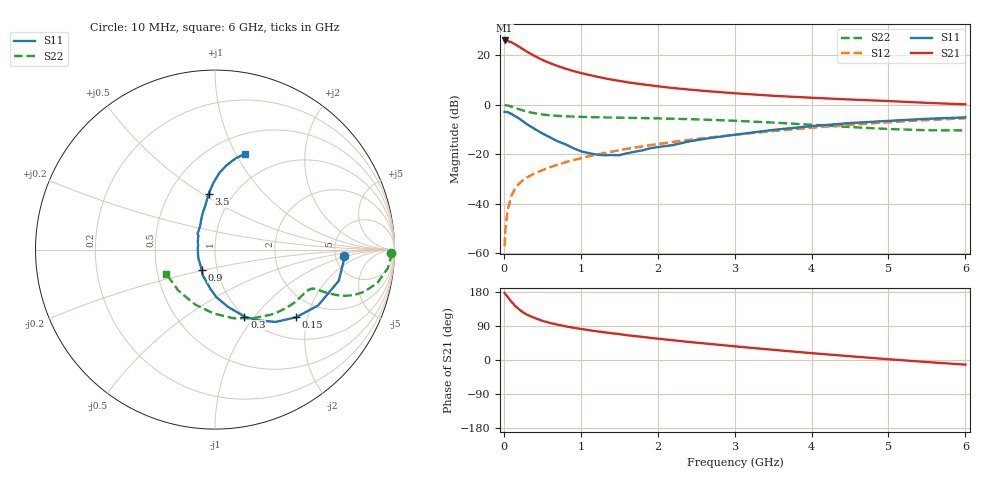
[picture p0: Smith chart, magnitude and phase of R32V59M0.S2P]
! SIEMENS Small Signal Semiconductors
! BFR181
! Si NPN RF Bipolar Junction Transistor in SOT23
! VCE = 2.5 V  IC = 9 mA
! Common Emitter S-Parameters:  May  1996
# GHz  S  MA  R  50
!  f  S11  S21  S12  S22
! GHz  MAG  ANG  MAG  ANG  MAG  ANG  MAG  ANG
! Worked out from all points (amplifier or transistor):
!   36 points, 10 MHz to 6 GHz, reference 50 ohm
!   highest |S21| = 26.0 dB at 10 MHz (marker M1)
!   |S21| within 3 dB of that: start of sweep to 222.1 MHz
!   unconditionally stable (mu >= 1): 777.7 MHz to 2.672 GHz
!   at 250 MHz: K = 0.59, MSG = 26.4 dB, |S12| = -30.4 dB
!   at 1.4 GHz: K = 1.07, MAG = 12.9 dB, |S12| = -18.9 dB
!   at 6 GHz: K = 0.85, MSG = 2.8 dB, |S12| = -5.4 dB
!   S11 on the Smith chart (normalised r, x): 10 MHz: 6.03, -0.95; 150 MHz: 1.47, -1.70; 300 MHz: 0.99, -0.89; 900 MHz: 0.84, -0.19; 3.5 GHz: 0.77, +0.53; 6 GHz: 0.70, +1.09
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0.01  0.7215 -3.0  19.93 177.1  0.0014 95.4  0.9834 -1.1
0.02  0.7178 -6.1  19.78 174.0  0.0031 86.6  0.9813 -2.6
0.05  0.7109 -14.2  19.43 166.2  0.0076 84.0  0.9674 -6.3
0.1  0.6533 -28.5  18.26 153.6  0.0147 77.8  0.9232 -11.6
0.15  0.5882 -39.9  16.49 142.0  0.0209 71.6  0.8669 -15.6
0.2  0.5259 -50.0  14.84 133.4  0.0257 70.1  0.8154 -18.1
0.25  0.4627 -58.5  13.24 125.7  0.0302 67.6  0.7681 -19.6
0.3  0.4075 -66.3  11.84 119.6  0.034 67.6  0.7292 -20.4
0.4  0.3259 -77.4  9.692 111.0  0.0414 67.1  0.6758 -21.1
0.5  0.265 -88.3  8.062 103.4  0.0477 67.6  0.639 -21.3
0.6  0.22 -96.9  6.933 97.8  0.055 68.2  0.6148 -21.2
0.7  0.1834 -105.5  6.071 93.1  0.0619 68.5  0.598 -21.5
0.9  0.1341 -123.7  4.823 85.2  0.0764 68.9  0.5792 -22.2
1.1  0.1062 -149.1  4.04 79.0  0.0913 69.5  0.5661 -23.5
1.3  0.0958 -171.8  3.454 73.3  0.1057 69.2  0.5569 -25.2
1.6  0.105 155.6  2.865 65.5  0.1288 68.5  0.5468 -28.3
2.2  0.1542 122.7  2.182 52.1  0.178 65.6  0.5235 -36.3
2.8  0.2261 106.5  1.808 40.0  0.2302 61.3  0.4907 -46.1
3.5  0.3115 96.6  1.523 26.9  0.2952 55.1  0.438 -60.8
4.5  0.4283 86.7  1.28 9.9  0.3953 44.0  0.3557 -91.4
5.5  0.5217 77.2  1.096 -5.4  0.4921 30.9  0.3065 -131.8
6  0.5571 72.8  1.021 -12.2  0.535 23.7  0.3041 -153.9
